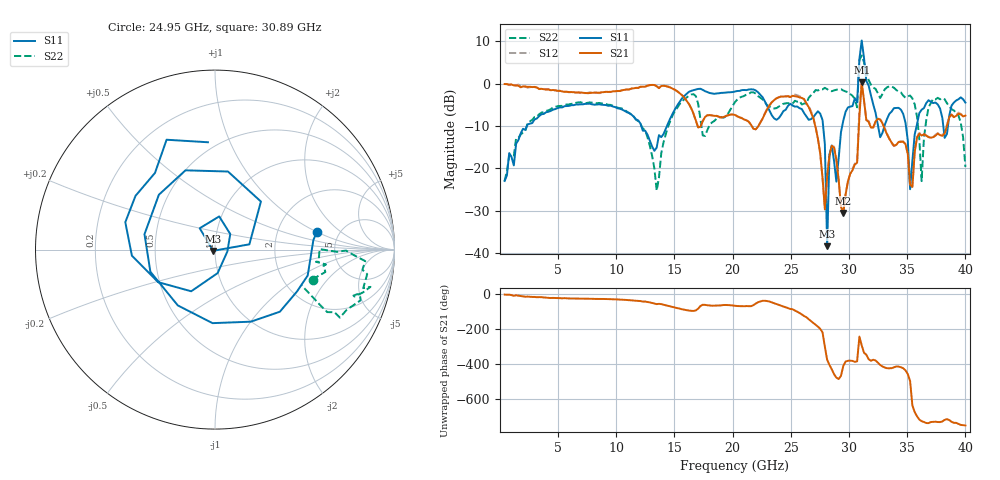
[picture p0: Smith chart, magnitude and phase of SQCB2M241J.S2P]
! Network Analyzer HP8722ES.07.66: Jul 25, 2000 Serial No. US39175408
! 27 Oct 2004  13:45:25
! Frequency  S11  S21  S12  S22
# HZ  S  DB R  50
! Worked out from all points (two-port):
!   201 points, 400 MHz to 40 GHz, reference 50 ohm
!   highest |S21| = 0.32 dB at 31.09 GHz (marker M1); lowest = -30.5 dB at 29.51 GHz (marker M2)
!   |S21| within 3 dB of the highest: start of sweep to 15.62 GHz; 31.02 GHz to 31.23 GHz (211.6 MHz wide, 0.68 % of centre)
!   lowest |S11| = -38.3 dB at 28.12 GHz (marker M3), VSWR 1.02, Z = 49 - j0.677 ohm
!   |S11| at or under -10 dB: start of sweep to 2.32 GHz; 12.15 GHz to 14.35 GHz (2.205 GHz wide, 16.6 % of centre); 27.77 GHz to 29.41 GHz (1.642 GHz wide, 5.74 % of centre)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
!   |S22| runs from -25.2 to 6.6 dB; largest |S21 - S12| = 0.13
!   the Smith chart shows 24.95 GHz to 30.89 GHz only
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4e8  -22.96 -99.4  -0.11 -2.5  -0.07 -2.0  -22.97 -98.3
7.132e9  -4.89 -98.7  -2.17 -25.2  -2.25 -26.1  -4.58 -129.8
1.3666e10  -12.16 -17.1  -1.09 -55.8  -1.03 -55.8  -22.19 125.3
1.6834e10  -1.41 4.5  -8.71 -93.6  -8.79 -94.2  -2.97 -69.8
2.02e10  -1.87 8.6  -7.39 -67.0  -7.41 -67.7  -4.36 -11.3
2.5546e10  -5.41 -15.6  -3.08 -100.8  -2.73 -101.8  -4.28 -8.3
2.6932e10  -7.91 167.7  -8.13 -164.6  -8.08 -166.6  -2.24 -2.2
2.7724e10  -8.63 46.3  -22.28 140.3  -22.42 138.6  -1.38 -14.6
2.812e10  -38.35 -145.2  -21.88 -17.2  -21.65 -18.0  -1.32 -16.1
2.8318e10  -16.69 125.6  -17.00 -46.2  -16.95 -46.4  -1.73 -18.6
2.9506e10  -8.75 -150.2  -30.52 -52.2  -30.51 -50.8  -1.64 -22.3
3.0694e10  -4.45 93.8  -18.68 -25.3  -18.53 -25.9  -5.62 -22.5
3.0892e10  5.77 52.1  -7.72 116.3  -5.37 119.5  5.61 -59.9
3.109e10  10.17 -88.1  0.32 65.7  0.04 65.0  6.62 -8.9
3.1486e10  0.62 -117.6  -8.60 12.5  -8.57 10.1  2.80 -27.1
3.1882e10  -2.77 -156.5  -10.36 -22.6  -10.27 -21.9  -0.28 -40.5
3.3466e10  -7.13 -139.8  -13.06 -65.4  -12.99 -64.6  -0.63 -27.6
3.4654e10  -7.14 177.7  -13.72 -65.2  -13.63 -65.8  -2.82 -51.8
3.5248e10  -24.92 167.1  -23.84 -138.4  -24.54 -141.5  -2.82 -58.3
3.6238e10  -6.17 -114.2  -12.27 -9.1  -12.00 -9.4  -23.00 -42.0
3.7228e10  -4.60 -138.8  -12.65 -12.6  -12.60 -13.0  -3.61 -23.2
4e10  -4.49 -133.8  -7.55 -33.4  -7.51 -33.6  -19.68 -120.4
